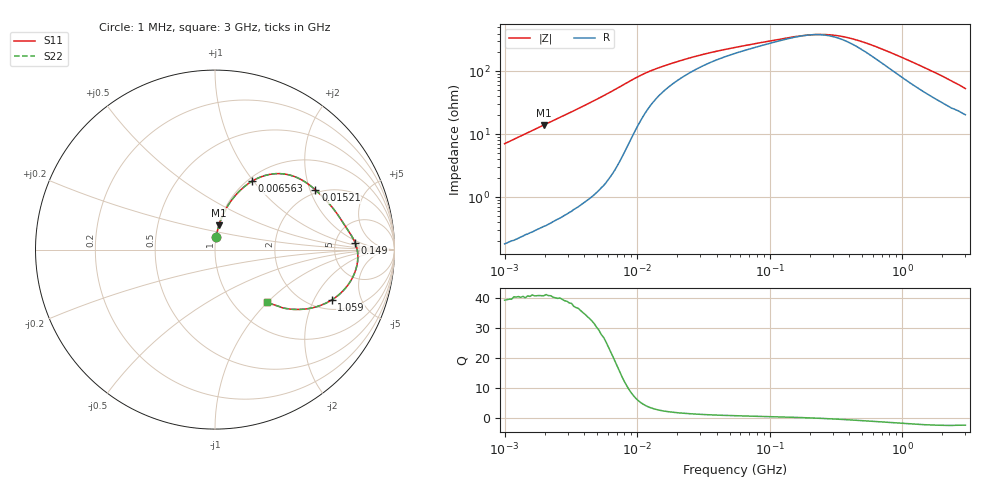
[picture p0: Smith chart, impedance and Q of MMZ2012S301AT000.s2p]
! S-parameter Generated by TDK Corporation
! Copyright(C) 2016 TDK Corporation.
! All Rights Reserved.
! TDK P/N: MMZ2012S301AT000 (Chip Beads)
! Property: |Z|=300¶ at 100MHz
! Size(LxWxT): 2x1.25x0.85mm, 0.079x0.049x0.033inches
! Model Type: s2p (Touchstone File Format Version 1.0)
! Frequency: DC=Yes Start=1MHz Stop=3000MHz 202points Log-sweep
! Note: This model was converted from impedance.
! Model Generated on May. 16, 2016
! Hash(MD5):
! Port Assignments:
!  1 ---@@@--- 2
! Applicable Conditions:
!  Temperature = 25 degC
!  DC Bias Current = 0 A
!  Small Signal Operation
! Terms and conditions regarding TDK Simulation Models
! (1)This simulation model is being provided solely for informational purposes. Please refer to the specifications of the products in terms of detailed characteristics of such products.
! (2)In no event shall TDK Corporation of any of its subsidiaries be liable for any loss or damage arising, directly or indirectly,
!  From any information contained in this simulation model, including, but not limited to loss or damages arising from any inaccuracies, omissions or errors in connection with such information.
! (3)Any and all copyrights on this simulation model are owned by TDK Corporation.
!  Duplication or redistribution of this simulation model without prior written permission from TDK Corporation is prohibited.
! (4)This simulation model is subject to any modification or change without any prior notice.
! (5)Neither TDK Corporation nor any of its subsidiaries shall make any warranty, express or implied,
!  Including but not limited to the correctness, implied warranties of merchantability and fitness for a particular purpose with respect to this simulation models.
! (6)The use of this simulation model shall be deemed to have consented to the terms and conditions hereof.
# MHz S MA R 50
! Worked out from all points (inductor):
!   201 points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, 1 MHz to 3 GHz, reference 50 ohm
!   read as one part in series: L = 1.13 uH near 1.041 MHz
!   highest Q = 40.7 at 1.975 MHz (marker M1), where L = 1.12 uH
!   self-resonance near 204.7 MHz
!   S11 on the Smith chart (normalised r, x): 1 MHz: 1.00, +0.14; 6.563 MHz: 1.05, +0.98; 15.21 MHz: 1.89, +2.18; 149 MHz: 7.88, +1.51; 1.059 GHz: 2.47, -2.78; 3 GHz: 1.41, -0.98
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1  0.07052 84.5  0.9957 -4.0  0.9957 -4.0  0.07052 84.5
1.974946  0.1378 80.7  0.9871 -7.9  0.9871 -7.9  0.1378 80.7
3.900413  0.2667 72.9  0.9562 -15.5  0.9562 -15.5  0.2667 72.9
5.161903  0.3479 67.7  0.9257 -20.3  0.9257 -20.3  0.3479 67.7
6.563319  0.4339 61.5  0.88 -25.7  0.88 -25.7  0.4339 61.5
8.017732  0.5118 54.6  0.8179 -30.7  0.8179 -30.7  0.5118 54.6
9.410094  0.5676 48.0  0.7503 -34.2  0.7503 -34.2  0.5676 48.0
11.49534  0.6151 39.8  0.6584 -36.7  0.6584 -36.7  0.6151 39.8
14.61624  0.6469 31.8  0.5648 -37.1  0.5648 -37.1  0.6469 31.8
15.21322  0.6508 30.7  0.5518 -37.0  0.5518 -37.0  0.6508 30.7
26.64524  0.6974 19.1  0.4101 -33.8  0.4101 -33.8  0.6974 19.1
54.77226  0.7363 10.5  0.3068 -25.9  0.3068 -25.9  0.7363 10.5
149.005  0.7819 2.7  0.2221 -9.7  0.2221 -9.7  0.7819 2.7
213.6344  0.7931 -0.4  0.207 1.5  0.207 1.5  0.7931 -0.4
282.7291  0.797 -3.2  0.209 12.3  0.209 12.3  0.797 -3.2
374.1707  0.7957 -6.4  0.2273 23.0  0.2273 23.0  0.7957 -6.4
558.3748  0.7806 -11.9  0.2857 34.3  0.2857 34.3  0.7806 -11.9
800.5644  0.7486 -18.0  0.3691 38.7  0.3691 38.7  0.7486 -18.0
1059.487  0.7075 -23.4  0.4497 38.7  0.4497 38.7  0.7075 -23.4
1855.641  0.5737 -35.5  0.6289 32.0  0.6289 32.0  0.5737 -35.5
2359.433  0.4955 -40.8  0.7042 27.4  0.7042 27.4  0.4955 -40.8
3000  0.4098 -45.2  0.7685 22.2  0.7685 22.2  0.4098 -45.2
